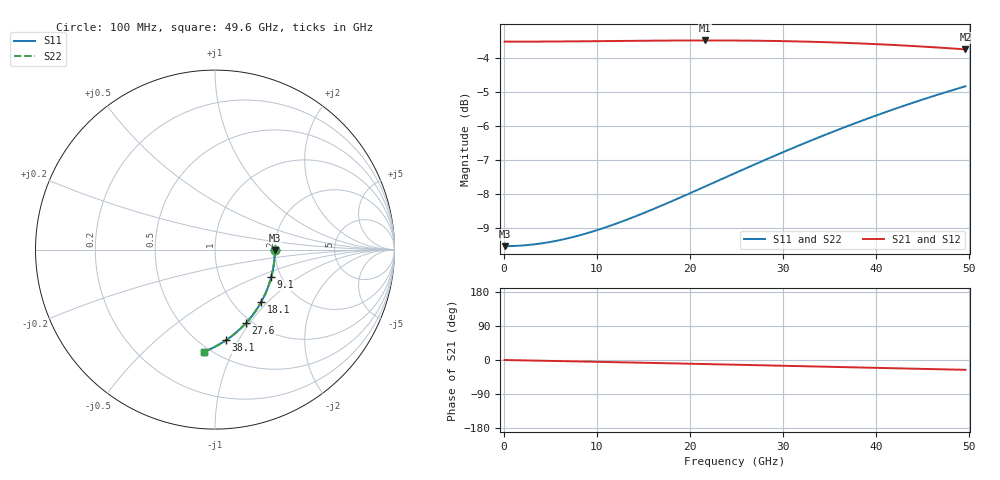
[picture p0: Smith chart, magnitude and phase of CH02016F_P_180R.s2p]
# GHz S RI R 180
! S-Parameters data
! Freq  reS11  imS11  reS21  imS21  reS12  imS12  reS22  imS22
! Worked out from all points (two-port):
!   100 points, 100 MHz to 49.6 GHz, reference 180 ohm
!   highest |S21| = -3.49 dB at 21.6 GHz (marker M1); lowest = -3.7 dB at 49.6 GHz (marker M2)
!   |S21| within 3 dB of the highest: start of sweep to end of sweep
!   lowest |S11| = -9.5 dB at 100 MHz (marker M3), VSWR 2.00, Z = 360 - j1.39 ohm
!   |S11| at or under -10 dB: nowhere
!   |S22| runs from -9.5 to -4.8 dB; largest |S21 - S12| = 0
!   S11 on the Smith chart (normalised r, x): 100 MHz: 2.00, -0.01; 9.1 GHz: 1.77, -0.62; 18.1 GHz: 1.34, -0.91; 27.6 GHz: 0.94, -0.96; 38.1 GHz: 0.66, -0.89; 49.6 GHz: 0.46, -0.78
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0.1  0.3333 -0.00171  0.6667 -0.000549  0.6667 -0.000549  0.3333 -0.00171
2.1  0.3322 -0.0359  0.6666 -0.0115  0.6666 -0.0115  0.3322 -0.0359
4.1  0.3292 -0.07  0.6665 -0.0226  0.6665 -0.0226  0.3292 -0.07
6.1  0.3243 -0.1037  0.6663 -0.0337  0.6663 -0.0337  0.3243 -0.1037
8.6  0.3154 -0.145  0.6658 -0.0477  0.6658 -0.0477  0.3154 -0.145
9.1  0.3133 -0.1532  0.6657 -0.0505  0.6657 -0.0505  0.3133 -0.1532
10.6  0.3064 -0.1773  0.6653 -0.059  0.6653 -0.059  0.3064 -0.1773
12.6  0.2957 -0.2088  0.6645 -0.0705  0.6645 -0.0705  0.2957 -0.2088
14.6  0.2833 -0.2393  0.6636 -0.0822  0.6636 -0.0822  0.2833 -0.2393
16.6  0.2696 -0.2687  0.6623 -0.094  0.6623 -0.094  0.2696 -0.2687
18.1  0.2584 -0.29  0.6612 -0.1029  0.6612 -0.1029  0.2584 -0.29
21.6  0.2296 -0.3371  0.6578 -0.124  0.6578 -0.124  0.2296 -0.3371
25.1  0.1977 -0.3801  0.6532 -0.1453  0.6532 -0.1453  0.1977 -0.3801
27.6  0.1733 -0.4083  0.6491 -0.1606  0.6491 -0.1606  0.1733 -0.4083
30.1  0.148 -0.4344  0.6443 -0.1757  0.6443 -0.1757  0.148 -0.4344
33.1  0.1166 -0.4629  0.6376 -0.1938  0.6376 -0.1938  0.1166 -0.4629
35.6  0.0898 -0.4844  0.6312 -0.2086  0.6312 -0.2086  0.0898 -0.4844
38.1  0.0626 -0.5038  0.6242 -0.223  0.6242 -0.223  0.0626 -0.5038
41.6  0.0243 -0.5278  0.6133 -0.2426  0.6133 -0.2426  0.0243 -0.5278
43.6  0.00232 -0.5399  0.6065 -0.2534  0.6065 -0.2534  0.00232 -0.5399
45.6  -0.0196 -0.5509  0.5994 -0.2639  0.5994 -0.2639  -0.0196 -0.5509
49.6  -0.0629 -0.5696  0.5842 -0.2838  0.5842 -0.2838  -0.0629 -0.5696
